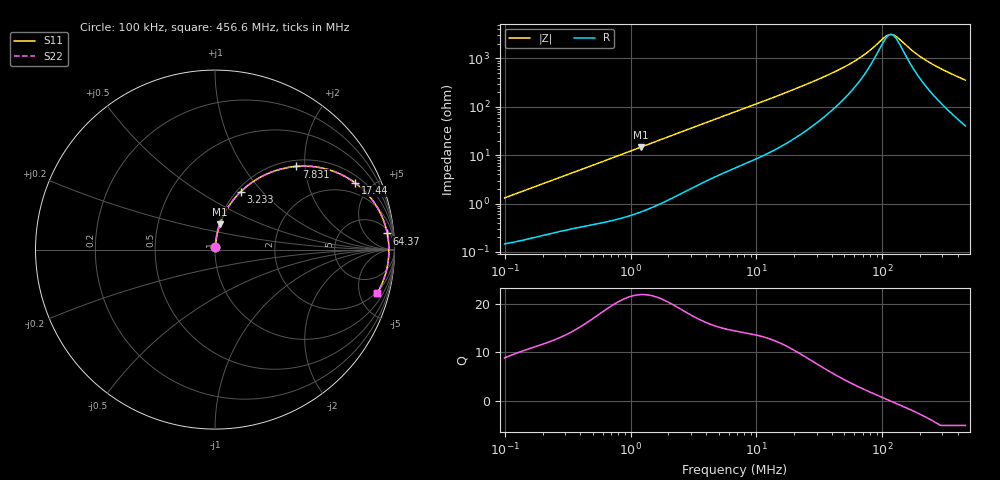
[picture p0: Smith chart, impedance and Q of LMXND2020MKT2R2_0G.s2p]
! LMXND2020MKT2R2_0G  S-PARAMETER MODEL  ( General Type )
! Model Generated by TAIYO YUDEN Corporation (https://www.yuden.co.jp/en/)
! Version 1.0
! TAIYO YUDEN Control No. 191023NI43SB-FBB
! Copyright(c) 2019 TAIYO YUDEN CO.,LTD. All Rights Reserved.
! Product Description (link to TY-COMPAS)
! https://ds.yuden.co.jp/TYCOMPAS/or/detail?pn=LMXND2020MKT2R2M0G&u=M
! Products Name : Inductors
! Characteristics :
!  Inductance : 2.2 uH , SRF(min) : -Hz , DC Resistance(max) : 0.1284 Ohm
!  Rated Current : Saturation :1350 mA , Temp Rise : 1370 mA (40 degC)
!  Case Size : 2.0 x 2.0 / 0.079 x 0.079 [mm/inch] , Thickness : 1.2 / 0.047 [mm/inch]
!  (Conditions: Temperature = 25 degC , DC Bias Current/Voltage = 0A / 0V)
! External Node Assignments :
!  1  o---GGG---o  2
! GND o---------o GND
! Frequency Range : 0.1MHz  -  456.598367MHz  [ 402 STEP ]
# MHz S RI R 50
! Freq[MHz].  S11 Real  S11 Imag  S21 Real  S21 Imag  S12 Real  S12 Imag  S22 Real  S22 Imag
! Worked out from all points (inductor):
!   401 points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, 100 kHz to 456.6 MHz, reference 50 ohm
!   read as one part in series: L = 2.06 uH near 104.3 kHz
!   highest Q = 21.9 at 1.201 MHz (marker M1), where L = 1.93 uH
!   self-resonance near 116.9 MHz
!   S11 on the Smith chart (normalised r, x): 100 kHz: 1.00, +0.03; 3.233 MHz: 1.04, +0.77; 7.831 MHz: 1.13, +1.80; 17.44 MHz: 1.35, +3.99; 64.37 MHz: 7, +19; 456.6 MHz: 1.81, -7.08
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0.1  0.00163 0.013  0.9984 -0.013  0.9984 -0.013  0.00163 0.013
0.410178  0.00585 0.0504  0.9942 -0.0504  0.9942 -0.0504  0.00585 0.0504
1.201054  0.0271 0.141  0.9729 -0.141  0.9729 -0.141  0.0271 0.141
1.682457  0.0481 0.1917  0.9519 -0.1917  0.9519 -0.1917  0.0481 0.1917
3.232644  0.1428 0.3221  0.8572 -0.3221  0.8572 -0.3221  0.1428 0.3221
4.723207  0.2489 0.4012  0.7511 -0.4012  0.7511 -0.4012  0.2489 0.4012
6.901063  0.3965 0.4556  0.6035 -0.4556  0.6035 -0.4556  0.3965 0.4556
7.830852  0.4524 0.4635  0.5476 -0.4635  0.5476 -0.4635  0.4524 0.4635
11.44163  0.6229 0.4482  0.3771 -0.4482  0.3771 -0.4482  0.6229 0.4482
17.43672  0.7808 0.3716  0.2192 -0.3716  0.2192 -0.3716  0.7808 0.3716
27.71655  0.8885 0.2597  0.1115 -0.2597  0.1115 -0.2597  0.8885 0.2597
44.99481  0.9423 0.1539  0.0577 -0.1539  0.0577 -0.1539  0.9423 0.1539
64.37135  0.96 0.0898  0.04 -0.0898  0.04 -0.0898  0.96 0.0898
79.46593  0.9654 0.0565  0.0346 -0.0565  0.0346 -0.0565  0.9654 0.0565
104.4999  0.9687 0.0161  0.0313 -0.0161  0.0313 -0.0161  0.9687 0.0161
113.6871  0.969 0.00398  0.031 -0.00398  0.031 -0.00398  0.969 0.00398
121.1038  0.969 -0.00508  0.031 0.00508  0.031 0.00508  0.969 -0.00508
129.0043  0.9689 -0.0142  0.0311 0.0142  0.0311 0.0142  0.9689 -0.0142
180.7114  0.9649 -0.0642  0.0351 0.0642  0.0351 0.0642  0.9649 -0.0642
237.6405  0.9568 -0.1092  0.0432 0.1092  0.0432 0.1092  0.9568 -0.1092
325.9515  0.9389 -0.1689  0.0611 0.1689  0.0611 0.1689  0.9389 -0.1689
456.5984  0.9033 -0.2441  0.0967 0.2441  0.0967 0.2441  0.9033 -0.2441
